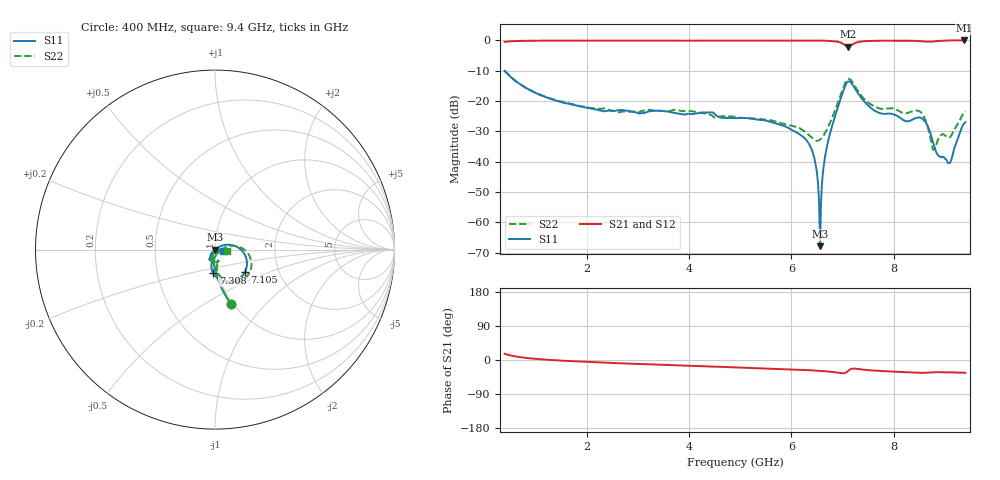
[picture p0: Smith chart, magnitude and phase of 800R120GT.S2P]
!  American Technical Ceramics  Date:  10/25/10
!  One Norden Lane
!  Huntington Station,  NY.  11746-2102
!  Tel:  (631) 622-4700  Fax:  (631) 622-4748
!  Part Number  800R120GT  Mounting Orientation: Vertical
!  Description: Ultra Low ESR Microwave Capacitor
!  Application: Coupling, Bypass, Tuning, DC Block, Filters, Matching
# GHZ S DB R 50
! Freq  |S11|  S11 Ph  |S21|  S21 Ph  |S12|  S12 Ph  |S22|  S22 Ph
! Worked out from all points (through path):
!   801 points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, 400 MHz to 9.4 GHz, reference 50 ohm
!   highest |S21| = -0.01 dB at 9.378 GHz (marker M1); lowest = -2.1 dB at 7.105 GHz (marker M2)
!   group delay of S21, straight-line fit = 12.9 ps
!   lowest |S11| = -67.9 dB at 6.565 GHz (marker M3), VSWR 1.00, Z = 50 + j0.0219 ohm
!   |S11| at or under -10 dB: start of sweep to end of sweep
!   |S22| runs from -36.1 to -10.0 dB; largest |S21 - S12| = 0.0015
!   S11 on the Smith chart (normalised r, x): 400 MHz: 0.98, -0.66; 7.105 GHz: 1.35, -0.35; 7.308 GHz: 0.95, -0.25; 9.4 GHz: 1.09, -0.02
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0.4  -10.00 -73.4  -0.46 16.6  -0.46 16.6  -9.97 -73.4
1.041  -17.58 -87.3  -0.09 2.6  -0.09 2.6  -17.55 -87.3
1.908  -21.88 -94.5  -0.05 -4.4  -0.05 -4.4  -21.74 -93.9
3.404  -23.20 -103.1  -0.04 -12.3  -0.04 -12.3  -23.20 -99.6
4.9  -25.64 -115.2  -0.04 -19.4  -0.04 -19.5  -25.26 -102.3
5.89  -28.43 -124.8  -0.05 -24.2  -0.05 -24.2  -27.67 -91.3
6.408  -36.43 -135.1  -0.03 -27.4  -0.03 -27.3  -32.14 -65.9
6.475  -40.98 -139.0  -0.03 -27.9  -0.03 -27.9  -33.01 -52.5
6.531  -49.77 -143.1  -0.04 -28.4  -0.04 -28.4  -33.02 -37.8
6.565  -67.89 32.8  -0.05 -28.8  -0.05 -28.8  -32.66 -28.5
6.599  -47.28 38.5  -0.07 -29.1  -0.06 -29.1  -32.05 -20.2
6.644  -39.98 36.7  -0.08 -29.5  -0.08 -29.5  -30.96 -10.1
6.711  -33.84 34.8  -0.11 -30.3  -0.12 -30.3  -28.80 1.9
7.105  -13.61 -37.1  -2.07 -29.3  -2.06 -29.3  -12.76 -31.7
7.308  -17.60 -94.2  -0.53 -23.8  -0.53 -23.8  -16.80 -80.6
7.904  -24.11 -97.4  -0.06 -30.1  -0.06 -30.0  -22.39 -72.8
8.568  -25.91 -115.4  -0.31 -33.9  -0.30 -33.9  -24.48 -97.6
8.781  -34.45 -130.1  -0.33 -32.2  -0.33 -32.2  -36.10 -70.2
8.928  -38.60 -86.8  -0.11 -32.2  -0.11 -32.2  -31.18 -37.4
9.074  -40.47 -47.1  -0.01 -32.8  0.00 -32.8  -32.10 -24.8
9.378  -27.33 -9.1  -0.01 -33.6  -0.01 -33.6  -23.71 -3.1
9.4  -27.00 -12.1  -0.01 -33.9  -0.01 -33.9  -23.32 -5.5
